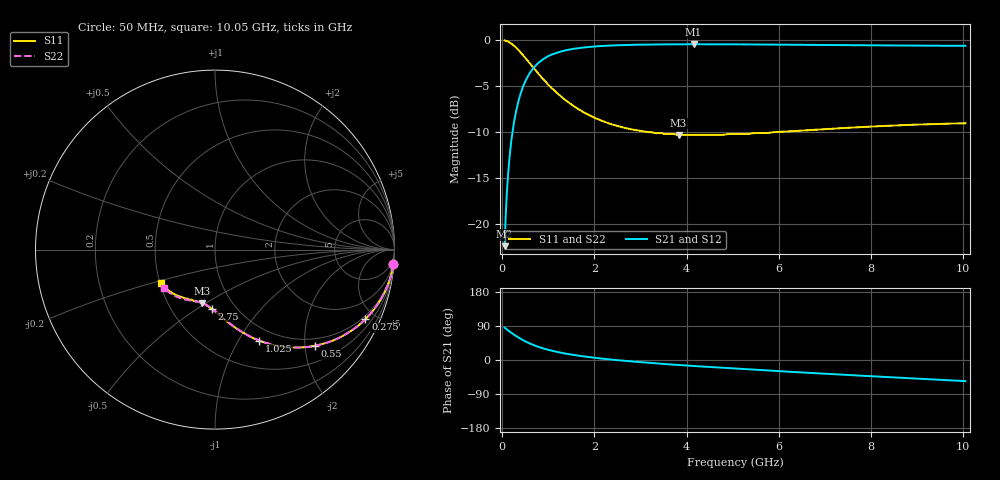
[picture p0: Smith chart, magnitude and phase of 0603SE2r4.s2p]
! AVX Thin Film Operation		Date: August 2001
! Description: Accu-P® Series, Thin Film, SMD, RF Capacitor
! Part Number: 06035J2R4ABT
! 50 MHz  -  10.05 GHz
! Serial Measurements
# mhz S db R 50
!	S11		S21		S12		S22
!	dB	Phase	dB	Phase	dB	Phase	dB	Phase
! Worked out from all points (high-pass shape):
!   401 points, 50 MHz to 10.05 GHz, reference 50 ohm
!   highest |S21| = -0.44 dB at 4.15 GHz (marker M1); lowest = -22.4 dB at 50 MHz (marker M2)
!   |S21| within 3 dB of the highest: 614.9 MHz to end of sweep
!   lowest |S11| = -10.3 dB at 3.825 GHz (marker M3), VSWR 1.88, Z = 36.7 - j24.1 ohm
!   |S11| at or under -10 dB: 3.2 GHz to 5.888 GHz (2.688 GHz wide, 59.1 % of centre)
!   |S22| runs from -10.3 to 0.0 dB; largest |S21 - S12| = 0
!   S11 on the Smith chart (normalised r, x): 50 MHz: 1, -24; 275 MHz: 0.83, -4.39; 550 MHz: 0.83, -2.22; 1.025 GHz: 0.83, -1.23; 2.75 GHz: 0.78, -0.57; 10.05 GHz: 0.51, -0.22
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50  -0.03 -4.8  -22.40 85.3  -22.40 85.3  -0.03 -4.8
75  -0.06 -7.1  -18.96 82.9  -18.96 82.9  -0.06 -7.1
125  -0.15 -11.7  -14.62 78.3  -14.62 78.3  -0.15 -11.7
150  -0.22 -14.0  -13.12 76.0  -13.12 76.0  -0.22 -14.0
200  -0.38 -18.5  -10.74 71.5  -10.74 71.5  -0.38 -18.5
275  -0.69 -24.8  -8.34 65.2  -8.34 65.2  -0.69 -24.8
325  -0.93 -28.8  -7.14 61.2  -7.14 61.2  -0.93 -28.8
400  -1.34 -34.3  -5.76 55.7  -5.76 55.7  -1.34 -34.3
550  -2.23 -43.8  -3.96 46.2  -3.96 46.2  -2.23 -43.8
775  -3.59 -54.9  -2.50 35.1  -2.50 35.1  -3.59 -54.9
1025  -4.97 -64.0  -1.67 25.9  -1.67 25.9  -4.97 -64.0
1350  -6.44 -72.6  -1.12 17.4  -1.12 17.4  -6.44 -72.5
1725  -7.71 -79.8  -0.81 10.2  -0.81 10.2  -7.71 -79.6
2175  -8.79 -86.6  -0.62 3.5  -0.62 3.5  -8.79 -86.2
2750  -9.64 -93.3  -0.51 -3.2  -0.51 -3.2  -9.63 -92.7
3400  -10.10 -99.7  -0.46 -9.5  -0.46 -9.5  -10.10 -98.9
3825  -10.30 -103.4  -0.44 -13.2  -0.44 -13.2  -10.24 -102.4
4150  -10.30 -106.0  -0.44 -15.8  -0.44 -15.8  -10.30 -105.0
5050  -10.20 -113.0  -0.45 -22.7  -0.45 -22.7  -10.20 -111.0
6725  -9.76 -126.0  -0.50 -34.3  -0.50 -34.3  -9.74 -122.0
8400  -9.29 -137.2  -0.57 -45.3  -0.57 -45.3  -9.27 -133.1
10050  -9.03 -147.8  -0.61 -55.7  -0.61 -55.7  -9.00 -142.8
